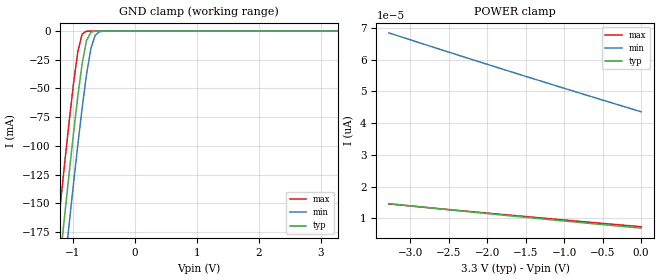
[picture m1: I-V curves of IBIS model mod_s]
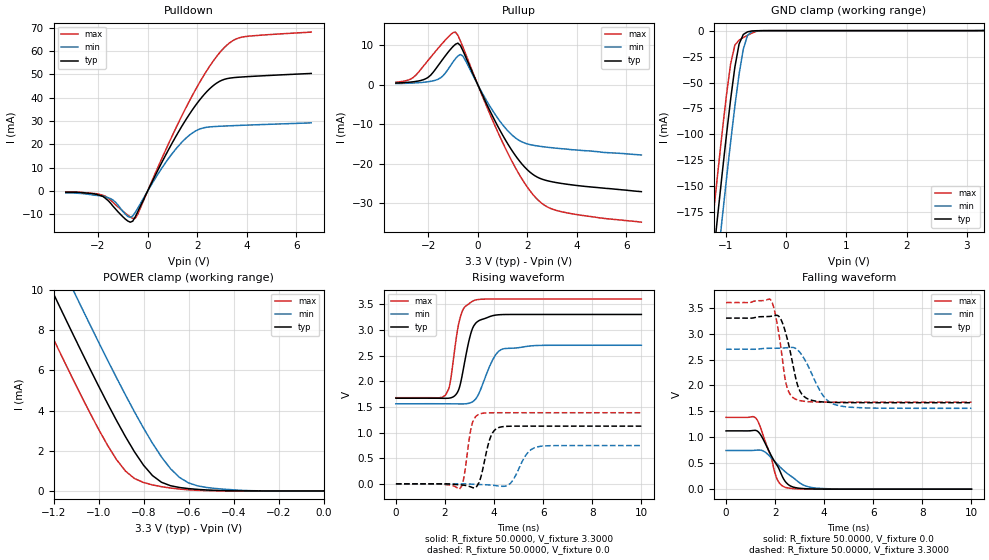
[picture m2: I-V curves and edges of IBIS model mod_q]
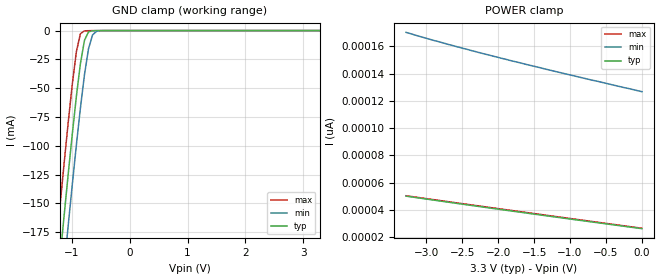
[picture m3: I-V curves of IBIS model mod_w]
| IBIS (I/O, Buffer, Information, Specification) Model, officially
| electronic behavioral standard for Buffer structures of digital pins.
[IBIS ver]  4.0
[File name] m95xxx_c5_tssop8.ibs
[File Rev]  1.0
[Date]   22 July 2016
[Source]   CAD & Design Services (Catania) - STMicroelectronics
[Notes]
   (Note1)  This IBIS model includes the TSSOP8 ceramic package parasitic data
   (Note2)  This IBIS model considers: VCC= 3.30(TYP), 2.70(MIN), 3.60(MAX)
   (Note3)  This IBIS model has some Notes about the non-monotonicity
   of the I-V curves, but they are not indicative of problems
   inside the model;
[Copyright] (c) 2016 STMicroelectronics
|   Component M95XXX
[Component] M95XXX
[Manufacturer] STMicroelectronics
[Package]
| variable   typ   min   max
R_pkg   0.0   0.0   0.0
L_pkg   0.0H   0.0H   0.0H
C_pkg   0.0F   0.0F   0.0F
[Pin]  signal_name   model_name   R_pin   L_pin   C_pin
1   SN   mod_s   NA   NA   NA
2   Q   mod_q   NA   NA   NA
3   WN   mod_w   NA   NA   NA
4   GND   GND   NA   NA   NA
5   D   mod_s   NA   NA   NA
6   C   mod_s   NA   NA   NA
7   HOLDN   mod_h   NA   NA   NA
8   VCCIO   POWER   NA   NA   NA
[Package Model]  182696_TSSOP8
[Define Package Model]  182696_TSSOP8
[Manufacturer]  STMicroelectronics
[OEM]  STMicroelectronics
[Description]  8 pin TSSOP package
[Number Of Pins]  8
[Pin Numbers]
|Pin Num   Terminal Name
1   | net1
2   | net2
3   | net3
4   | net4_GND
5   | net5
6   | net6
7   | net7
8   | net8_VDD
[Model Data]
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[End Model Data]
[End Package Model]
| Models and submodels in the file (4): mod_s (Input), mod_q (I/O), mod_w (Input), mod_h (Input)
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|   Model mod_s
[Model]   mod_s
Model_type Input
Vinl   =   0.825V
Vinh   =   2.475V
C_comp   2.119pF   2.024pF   2.324pF
[Temperature Range]  25.0000   85.0000   -40.0000
[Voltage Range]   3.3000V   2.7000V   3.6000V
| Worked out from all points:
|   GND clamp passes 1 mA (typ) near -0.70 V on its own axis
[GND_clamp]
|Voltage   I(typ)   I(min)   I(max)
-3.3V     -1.355A    -1.397A    -1.313A
-1.27V    -233mA     -277.9mA   -187.4mA
-1.2V     -196.1mA   -241mA     -150.5mA
-1.13V    -159.7mA   -204.5mA   -114.2mA
-1.06V    -124.1mA   -168.5mA   -79.16mA
-920mV    -57.12mA   -99.32mA   -18.15mA
-850mV    -28.51mA   -67.14mA   -2.609mA
-780mV    -8.357mA   -38.23mA   -131.1uA
-710mV    -1.089mA   -15.64mA   -5.451uA
-640mV    -95.71uA   -3.67mA    -224.5nA
-570mV    -7.943uA   -542uA     -9.245nA
3.28V     6.871pA    47.88pA    6.69pA
[POWER_clamp]
|Voltage   I(typ)   I(min)   I(max)
-3.28V    14.67pA    68.47pA    14.54pA
-2.48V    12.67pA    62.23pA    12.73pA
-1.72V    10.84pA    56.42pA    11.05pA
0V        6.915pA    43.6pA     7.361pA
|   Model mod_q
[Model]   mod_q
Model_type I/O
Polarity   Non-Inverting
Enable   Active-Low
Vinl   =   0.825V
Vinh   =   2.475V
Vmeas  =   1.650V
Cref   =   30pF
C_comp   2.793pF   2.547pF   2.925pF
[Temperature Range]  25.0000   85.0000   -40.0000
[Voltage Range]   3.3000V   2.7000V   3.6000V
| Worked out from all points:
|   slope of the pulldown table from 0 to 0.495 V, typ, clamps not added: 46.4 ohm
|   slope of the pullup table from 0 to 0.495 V, typ, clamps not added: 74.4 ohm
|   GND clamp passes 1 mA (typ) near -0.63 V on its own axis
|   POWER clamp passes 1 mA (typ) near -0.78 V on its own axis
|   rising waveform, R_fixture 50.0000, V_fixture 3.3000: 20-80 % time 433ps typ, 604ps min, 364ps max; typ from 1.67 V to 3.3 V
|   rising waveform, R_fixture 50.0000, V_fixture 0.0: 20-80 % time 338ps typ, 496ps min, 253ps max; typ from 0 V to 1.12 V
|   falling waveform, R_fixture 50.0000, V_fixture 0.0: 20-80 % time 734ps typ, 1.06ns min, 550ps max; typ from 1.12 V to 0 V
|   falling waveform, R_fixture 50.0000, V_fixture 3.3000: 20-80 % time 470ps typ, 743ps min, 362ps max; typ from 3.3 V to 1.67 V
[Pulldown]
|Voltage   I(typ)   I(min)   I(max)
-3.3V     -468uA     -780uA     -402uA
-1.7V     -3.1mA     -2.5mA     -2.2mA
-1.3V     -7.6mA     -4.7mA     -5.8mA
-800mV    -12.81mA   -10.84mA   -10.31mA
-600mV    -12.87mA   -10.65mA   -11.67mA
-500mV    -11.06mA   -9.142mA   -11.69mA
600mV     12.83mA    10.26mA    14.6mA
1.5V      29.85mA    22.21mA    34.77mA
2.3V      41.61mA    27.2mA     50.15mA
3V        47.52mA    27.83mA    60.44mA
3.8V      48.9mA     28.19mA    65.96mA
6.6V      50.42mA    29.25mA    68.14mA
[Pullup]
|Voltage   I(typ)   I(min)   I(max)
-3.3V     396uA      256uA      605uA
-2.6V     716uA      408uA      1.803mA
-2V       1.843mA    727uA      6.14mA
-1.4V     6.505mA    2.229mA    10.62mA
-900mV    10.2mA     6.549mA    13.29mA
-600mV    8.618mA    7.238mA    9.547mA
400mV     -5.428mA   -4.518mA   -6.111mA
1.2V      -14.87mA   -11.6mA    -17.18mA
1.8V      -20.21mA   -14.54mA   -24.03mA
2.4V      -23.39mA   -15.51mA   -28.99mA
3.4V      -25.02mA   -16.22mA   -32.17mA
6.6V      -27.08mA   -17.8mA    -34.8mA
[GND_clamp]
|Voltage   I(typ)   I(min)   I(max)
-3.3V     -1.447A    -1.488A    -1.41A
-1.27V    -253.6mA   -297.1mA   -213.1mA
-1.2V     -214.3mA   -257.8mA   -173.7mA
-1.13V    -175.5mA   -219mA     -135.1mA
-1.06V    -137.5mA   -180.7mA   -97.61mA
-920mV    -65.95mA   -107.1mA   -31.83mA
-850mV    -35.13mA   -72.81mA   -13.93mA
-780mV    -12.87mA   -41.97mA   -9.13mA
-710mV    -3.674mA   -17.74mA   -6.723mA
-640mV    -1.164mA   -4.638mA   -4.512mA
-430mV    -26.5uA    -95.56uA   -68.17uA
3.28V     150.3pA    314.7uA    122.1pA
[POWER_clamp]
|Voltage   I(typ)   I(min)   I(max)
-3.28V    60.68mA    62.78mA    58.54mA
-1.32V    12.64mA    14.86mA    10.38mA
-1.28V    11.69mA    13.91mA    9.431mA
-1.2V     9.805mA    12.03mA    7.55mA
-1.12V    7.943mA    10.16mA    5.704mA
-1.08V    7.024mA    9.234mA    4.803mA
-960mV    4.351mA    6.513mA    2.274mA
-880mV    2.694mA    4.768mA    984.9uA
-760mV    761.3uA    2.37mA     298.5uA
-640mV    170.6uA    670.6uA    92.55uA
-480mV    28.08uA    121.3uA    6.586uA
0V        154.1pA    603.1pA    158pA
[Ramp]
| variable   typ   min   max
dV/dt_r  0.6746/0.3725n   0.4473/0.5402n   0.8315/0.3057n
dV/dt_f  0.9785/0.5219n   0.6838/0.8293n   1.1512/0.4317n
R_load = 50.0000
[Rising Waveform]
R_fixture= 50.0000
V_fixture= 3.3000
V_fixture_min= 2.7000
V_fixture_max= 3.6000
|time   V(typ)   V(min)   V(max)
0s        1.668V     1.56V      1.678V
2.03ns    1.666V     1.56V      1.736V
2.21ns    1.673V     1.559V     1.971V
2.49ns    1.77V      1.558V     2.939V
2.63ns    1.955V     1.557V     3.258V
2.97ns    2.775V     1.57V      3.507V
3.17ns    3.076V     1.615V     3.569V
3.95ns    3.277V     2.424V     3.6V
4.31ns    3.297V     2.62V      3.6V
10ns      3.3V       2.7V       3.6V
[Rising Waveform]
R_fixture= 50.0000
V_fixture= 0.0
V_fixture_min= 0.0
V_fixture_max= 0.0
|time   V(typ)   V(min)   V(max)
0s        5.492nV    45.04nV    5.446nV
2.59ns    -18.73mV   118.2uV    -103.9mV
2.77ns    -26.35mV   -940.8uV   126.7mV
3.09ns    -67.03mV   -6.257mV   1.141V
3.43ns    82.31mV    -14.13mV   1.365V
3.83ns    877.7mV    -23.12mV   1.384V
4.17ns    1.093V     -40.92mV   1.385V
4.67ns    1.123V     10.28mV    1.385V
5.75ns    1.124V     718.4mV    1.385V
10ns      1.124V     745.6mV    1.385V
[Falling Waveform]
R_fixture= 50.0000
V_fixture= 0.0
V_fixture_min= 0.0
V_fixture_max= 0.0
|time   V(typ)   V(min)   V(max)
0s        1.124V     745.6mV    1.385V
1.22ns    1.132V     751.9mV    1.366V
1.43ns    1.033V     750.2mV    1.155V
1.81ns    677mV      622.1mV    654.4mV
2.07ns    465.5mV    492mV      204.9mV
2.25ns    289.2mV    405.2mV    80.03mV
2.46ns    121.2mV    316.2mV    28.76mV
3.13ns    12.12mV    83.63mV    2.877mV
3.73ns    2.65mV     18.1mV     387.1uV
10ns      -30.59nV   280.1nV    -17.72nV
[Falling Waveform]
R_fixture= 50.0000
V_fixture= 3.3000
V_fixture_min= 2.7000
V_fixture_max= 3.6000
|time   V(typ)   V(min)   V(max)
0s        3.3V       2.7V       3.6V
1.81ns    3.334V     2.718V     3.659V
2.06ns    3.354V     2.719V     3.248V
2.25ns    3.26V      2.721V     2.675V
2.47ns    2.944V     2.728V     1.992V
2.87ns    2.081V     2.704V     1.728V
3.25ns    1.762V     2.463V     1.692V
3.97ns    1.682V     1.795V     1.679V
4.45ns    1.672V     1.63V      1.678V
10ns      1.668V     1.56V      1.678V
|   Model mod_w
[Model]   mod_w
Model_type Input
Vinl   =   0.825V
Vinh   =   2.475V
C_comp   2.119pF   2.024pF   2.324pF
[Temperature Range]  25.0000   85.0000   -40.0000
[Voltage Range]   3.3000V   2.7000V   3.6000V
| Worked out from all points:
|   GND clamp passes 1 mA (typ) near -0.70 V on its own axis
[GND_clamp]
|Voltage   I(typ)   I(min)   I(max)
-3.3V     -1.356A    -1.398A    -1.314A
-1.27V    -233.3mA   -278.1mA   -187.7mA
-1.2V     -196.3mA   -241.2mA   -150.7mA
-1.13V    -159.9mA   -204.7mA   -114.5mA
-1.06V    -124.2mA   -168.7mA   -79.35mA
-920mV    -57.23mA   -99.42mA   -18.3mA
-850mV    -28.6mA    -67.22mA   -2.741mA
-780mV    -8.432mA   -38.3mA    -241.4uA
-710mV    -1.144mA   -15.69mA   -94.22uA
-640mV    -132.4uA   -3.703mA   -67.87uA
-570mV    -28.85uA   -563.3uA   -47.22uA
3.28V     26.19pA    133.9pA    24.34pA
[POWER_clamp]
|Voltage   I(typ)   I(min)   I(max)
-3.28V    50.17pA    170.3pA    50.46pA
-2.68V    45.65pA    161.3pA    46.01pA
-1.84V    39.47pA    149.8pA    39.87pA
-1.32V    35.7pA     143.1pA    36.1pA
0V        26.33pA    126.8pA    26.62pA
